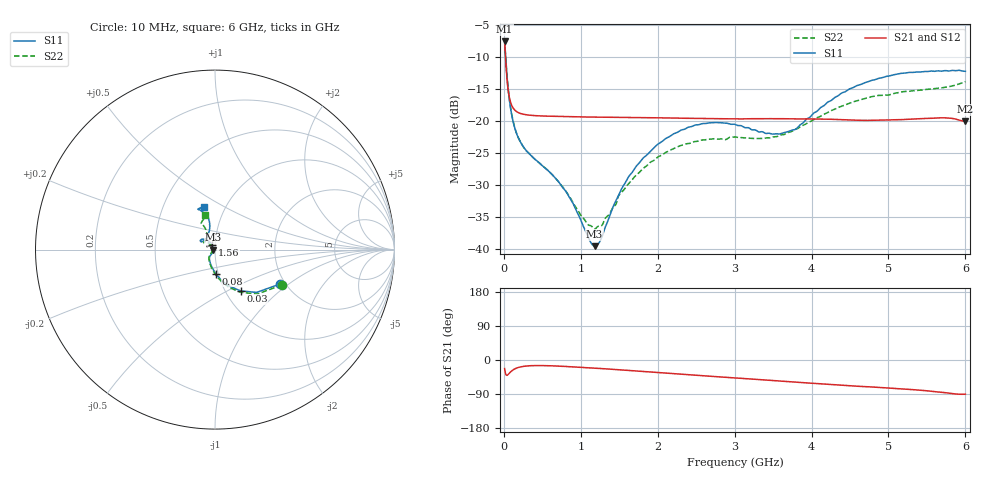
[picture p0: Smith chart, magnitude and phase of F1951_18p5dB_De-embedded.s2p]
! Integrated Device Technology
! Corporate Headquarters
! 6024 Silver Creek Valley Road
! San Jose, CA 95138  USA
! Phone:  1-408-284-8200
! Toll Free:  1-800-223-1366
! Webpage:  http://www.idt.com/
! Timing and RF Division
! 515 Groton Road, Suite 102
! Westford, MA 01886-6024
! Device:  F1951
! Description: 6-bit 0.5 dB Digital Step Attenuator
! Frequency:  100.0 -  4000.00 MHz
! Package:  4x4 mm Thin QFN Plastic Package: 24 pin
! Ports:  2 RF, 6 DC
!  Pin  1  = NC
!  Pin  2  = RF1  =  Port 1
!  Pin  3  = GND
!  Pin  4  = NC
!  Pin  5  = Serial Data Out (SDO)
!  Pin  6  = NC
!  Pin  7  = Reset Bar ( RSTb)
!  Pin  8  = Clock (CLK)
!  Pin  9  = Chip Select Bar (CSb)
!  Pin 10  = NC
!  Pin 11  = Serial Data In (SDI)
!  Pin 12  = NC
!  Pin 13  = NC
!  Pin 14  = VDD
!  Pin 15  = NC
!  Pin 16  = GND
!  Pin 17  = RF2  =  Port 2
!  Pin 18  = NC
!  Pin 19  = GND
!  Pin 20  = GND
!  Pin 21  = GND
!  Pin 22  = GND
!  Pin 23  = GND
!  Pin 24  = GND
! State:  37
! Atten State:  18.5 dB
! Voltage:  +3.30 Volts
! Current:  0.489 mA
! Data:  The device was measured on a F195X evaluation board which has
!  individual transmission lines to the RF pins.  Data was collected
!  de-embedded using a Automatic Fixture Removal [AFR] (Keysight Technologies).
!  The reference plane is the edge of the package pin.
! Misc:  Lot Code  1225BCA
!  Action Tracker AT0399
! Date Measured:  2018-09-13
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# GHz S dB R 50
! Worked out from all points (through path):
!   600 points, 10 MHz to 6 GHz, reference 50 ohm
!   highest |S21| = -7.63 dB at 10 MHz (marker M1); lowest = -20.1 dB at 6 GHz (marker M2)
!   group delay of S21, straight-line fit = 36 ps
!   lowest |S11| = -39.6 dB at 1.18 GHz (marker M3), VSWR 1.02, Z = 49 + j0.00464 ohm
!   |S11| at or under -10 dB: 22.41 MHz to end of sweep
!   |S22| runs from -36.9 to -7.5 dB; largest |S21 - S12| = 0.00027
!   S11 on the Smith chart (normalised r, x): 10 MHz: 1.88, -0.87; 30 MHz: 1.18, -0.58; 80 MHz: 0.97, -0.27; 1.56 GHz: 0.96, +0.05; 6 GHz: 0.80, +0.40
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0.01  -7.73 -27.8  -7.63 -22.5  -7.63 -22.5  -7.48 -27.7
0.03  -11.37 -58.3  -11.71 -39.6  -11.71 -39.7  -11.18 -59.3
0.05  -14.34 -74.1  -14.60 -39.4  -14.60 -39.5  -14.22 -75.5
0.08  -17.46 -88.1  -16.80 -33.1  -16.80 -33.1  -17.38 -90.0
0.15  -21.45 -106.7  -18.43 -22.7  -18.42 -22.7  -21.41 -108.7
0.25  -23.99 -119.3  -18.98 -17.0  -18.98 -16.9  -24.02 -122.3
0.71  -29.48 -127.8  -19.33 -16.1  -19.32 -16.1  -29.52 -136.5
0.87  -32.29 -129.9  -19.37 -17.8  -19.37 -17.8  -32.14 -141.1
1.01  -35.78 -138.3  -19.41 -19.4  -19.41 -19.4  -34.89 -150.2
1.18  -39.56 179.7  -19.43 -21.4  -19.43 -21.4  -36.87 -178.2
1.26  -38.53 152.7  -19.43 -22.4  -19.43 -22.4  -36.42 166.5
1.56  -30.04 123.0  -19.47 -26.5  -19.47 -26.5  -30.78 134.9
1.79  -26.11 123.7  -19.50 -29.9  -19.50 -29.9  -27.67 132.3
2.01  -23.60 129.1  -19.54 -33.1  -19.54 -33.1  -25.59 134.9
2.49  -20.66 141.2  -19.63 -40.1  -19.63 -40.1  -23.24 142.6
3.01  -20.59 150.5  -19.70 -47.4  -19.70 -47.4  -22.53 146.3
3.59  -22.05 129.9  -19.68 -55.6  -19.68 -55.6  -22.25 128.8
3.79  -21.35 115.7  -19.72 -58.4  -19.72 -58.4  -21.33 122.1
4.01  -19.03 105.9  -19.72 -61.6  -19.72 -61.5  -19.97 116.6
4.49  -15.06 101.7  -19.87 -68.1  -19.87 -68.0  -17.28 114.8
5.01  -13.02 108.9  -19.88 -73.8  -19.88 -73.8  -15.97 117.5
6  -12.29 104.7  -20.10 -90.2  -20.10 -90.2  -13.90 106.5
